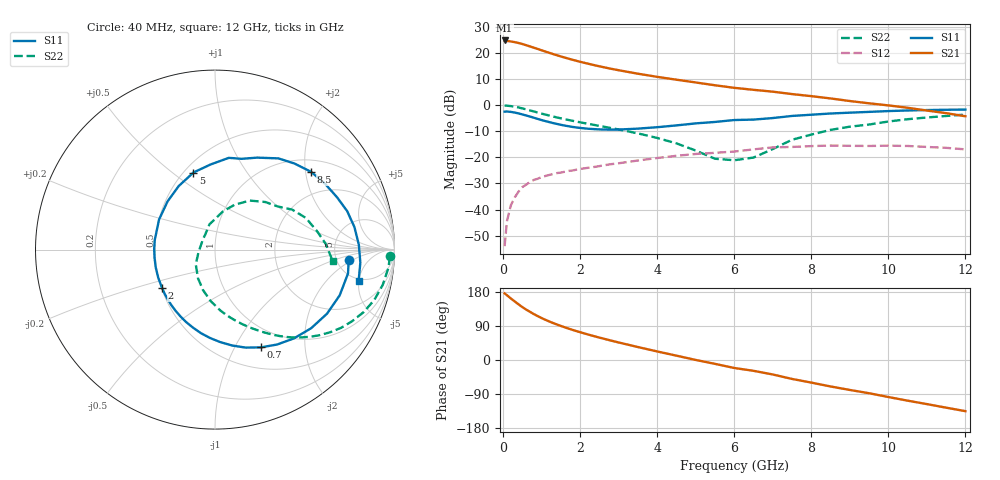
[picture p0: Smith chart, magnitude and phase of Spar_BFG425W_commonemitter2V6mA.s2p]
! Filename: 26bfg425.001
! BFG425W Field C1
! V1=8.342E-001V,V2=2.000E+000V, I1=7.965E-005A, I2=6.010E-003A
# GHz  S  MA  R 50
!  S11  S21  S12  S22
!Freq(GHz)  Mag  Ang  Mag  Ang  Mag  Ang  Mag  Ang
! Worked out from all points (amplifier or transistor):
!   44 points, 40 MHz to 12 GHz, reference 50 ohm
!   highest |S21| = 24.7 dB at 40 MHz (marker M1)
!   |S21| within 3 dB of that: start of sweep to 847.2 MHz
!   unconditionally stable (mu >= 1): 2.286 GHz to end of sweep
!   at 700 MHz: K = 0.38, MSG = 25.9 dB, |S12| = -29.4 dB
!   at 2.4 GHz: K = 1.03, MAG = 18.3 dB, |S12| = -23.6 dB
!   at 12 GHz: K = 1.46, MAG = 2.3 dB, |S12| = -17.0 dB
!   S11 on the Smith chart (normalised r, x): 40 MHz: 6.47, -1.66; 700 MHz: 0.75, -1.28; 2 GHz: 0.50, -0.25; 5 GHz: 0.56, +0.60; 8.5 GHz: 1.31, +2.15; 12 GHz: 4.68, -4.96
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0.04  0.747 -4.4  17.19 175.8  0.002 73.9  0.975 -2.2
0.1  0.753 -10.1  16.82 171.0  0.006 84.3  0.972 -5.9
0.2  0.74 -20.1  16.45 162.5  0.012 78.2  0.955 -11.9
0.3  0.719 -29.8  15.97 154.7  0.017 73.5  0.931 -17.5
0.4  0.692 -39.3  15.37 147.0  0.022 68.3  0.899 -22.7
0.5  0.662 -48.4  14.71 139.6  0.027 63.8  0.863 -27.5
0.6  0.632 -56.8  13.95 133.0  0.03 59.9  0.827 -31.8
0.7  0.602 -64.8  13.2 127.0  0.034 56.3  0.789 -35.7
0.8  0.572 -72.7  12.5 121.1  0.037 53.3  0.753 -39.3
1  0.516 -86.8  11.15 110.7  0.042 48.4  0.686 -45.5
1.3  0.452 -105.7  9.434 97.5  0.048 43.0  0.603 -53.1
1.6  0.405 -123.0  8.091 86.3  0.053 39.2  0.537 -59.3
2  0.365 -143.7  6.727 73.4  0.06 35.4  0.468 -66.7
2.2  0.353 -153.6  6.188 67.5  0.063 33.7  0.439 -70.3
3  0.34 170.8  4.633 46.3  0.077 27.0  0.341 -84.9
3.5  0.354 151.6  3.978 34.2  0.087 22.0  0.287 -95.0
4.5  0.408 119.6  3.053 11.4  0.107 10.3  0.185 -120.9
5  0.446 105.6  2.705 0.1  0.116 2.7  0.135 -142.5
6.5  0.527 73.7  1.956 -28.6  0.142 -13.6  0.099 123.9
8.5  0.689 38.9  1.338 -69.8  0.168 -49.2  0.335 54.6
10.5  0.787 9.1  0.887 -107.3  0.165 -83.9  0.536 19.2
12  0.819 -12.3  0.61 -135.0  0.142 -113.8  0.658 -5.5
